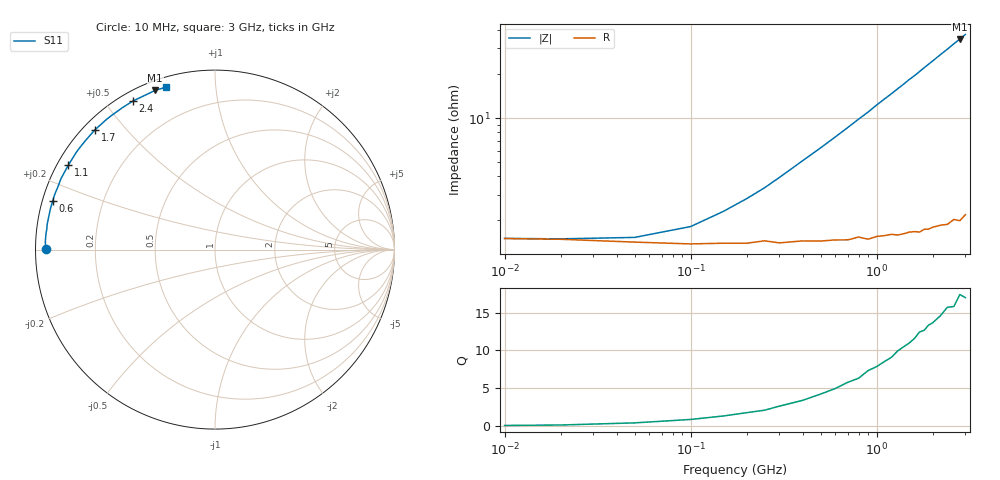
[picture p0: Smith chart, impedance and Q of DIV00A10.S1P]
! SIEMENS Small Signal Semiconductors
! BAV99
! Silicon Switching Diode in SOT23
! IF = 100 mA
! S-Parameters:  May  1995
# GHz  S  MA  R  50
!  f  S11
! GHz  MAG  ANG
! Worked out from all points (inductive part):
!   30 points, 10 MHz to 3 GHz, reference 50 ohm
!   read as one part to ground: L = 1.94 nH near 400 MHz
!   highest Q = 17 at 2.8 GHz (marker M1), where L = 1.97 nH
!   S11 on the Smith chart (normalised r, x): 10 MHz: 0.03, +0.00; 600 MHz: 0.03, +0.15; 1.1 GHz: 0.03, +0.27; 1.7 GHz: 0.03, +0.41; 2.4 GHz: 0.04, +0.59; 3 GHz: 0.04, +0.74
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0.01  0.9416 179.8
0.02  0.9423 179.6
0.05  0.9447 178.7
0.1  0.9463 177.3
0.15  0.9457 175.8
0.2  0.9458 174.4
0.25  0.9438 173.1
0.3  0.9457 171.6
0.4  0.9442 168.8
0.5  0.9446 166.1
0.6  0.944 163.4
0.7  0.9444 160.7
0.8  0.9424 158.0
0.9  0.9448 155.4
1  0.9431 152.6
1.1  0.943 150.0
1.2  0.9425 147.5
1.3  0.9438 144.9
1.4  0.9435 142.4
1.5  0.943 139.8
1.6  0.9434 137.5
1.7  0.9447 135.0
1.9  0.9443 130.1
2.2  0.9442 123.2
2.4  0.9458 118.9
2.6  0.9441 114.6
2.8  0.9476 110.6
3  0.9452 106.7
